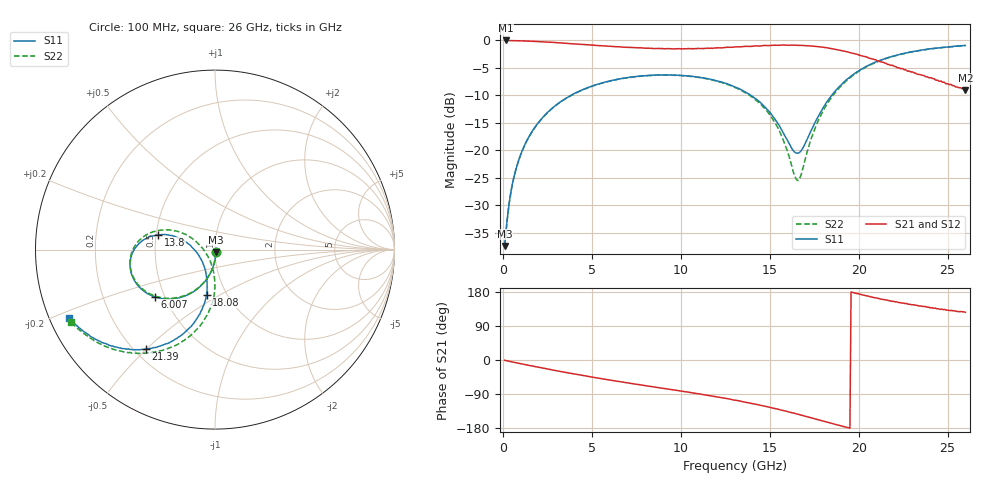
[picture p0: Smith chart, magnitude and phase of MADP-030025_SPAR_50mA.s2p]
!Mean
# HZ S DB R 50
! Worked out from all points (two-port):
!   400 points, 100 MHz to 26 GHz, reference 50 ohm
!   highest |S21| = -0.03 dB at 164.9 MHz (marker M1); lowest = -9.1 dB at 26 GHz (marker M2)
!   |S21| within 3 dB of the highest: start of sweep to 20.44 GHz
!   lowest |S11| = -37.4 dB at 100 MHz (marker M3), VSWR 1.03, Z = 50.4 - j1.29 ohm
!   |S11| at or under -10 dB: start of sweep to 3.835 GHz; 13.94 GHz to 18.49 GHz (4.546 GHz wide, 28 % of centre)
!   |S22| runs from -37.4 to -0.9 dB; largest |S21 - S12| = 0.0063
!   S11 on the Smith chart (normalised r, x): 100 MHz: 1.01, -0.03; 6.007 GHz: 0.44, -0.28; 13.8 GHz: 0.51, +0.09; 18.08 GHz: 0.81, -0.43; 21.39 GHz: 0.25, -0.50; 26 GHz: 0.06, -0.22
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1e8  -37.38 -71.7  -0.04 -0.8  -0.04 -0.8  -37.41 -71.7
1.6491e8  -35.34 -76.2  -0.03 -1.6  -0.04 -1.5  -35.26 -76.8
3.5965e8  -29.53 -84.0  -0.05 -3.5  -0.05 -3.5  -29.55 -84.1
5.5439e8  -25.86 -88.6  -0.06 -5.4  -0.07 -5.4  -25.93 -88.4
1.3333e9  -18.32 -99.5  -0.13 -12.9  -0.14 -12.9  -18.38 -99.6
2.6316e9  -12.75 -112.9  -0.34 -24.9  -0.34 -24.9  -12.79 -113.3
4.4491e9  -9.03 -129.4  -0.75 -40.6  -0.75 -40.6  -9.06 -130.0
6.007e9  -7.40 -142.0  -1.09 -53.0  -1.10 -53.0  -7.42 -142.8
8.7982e9  -6.30 -162.3  -1.47 -73.3  -1.48 -73.3  -6.34 -163.7
1.1005e10  -6.69 -177.1  -1.47 -89.1  -1.47 -89.1  -6.74 -179.5
1.3082e10  -8.52 169.3  -1.20 -106.2  -1.22 -106.2  -8.62 165.3
1.3796e10  -9.70 165.4  -1.11 -112.6  -1.11 -112.7  -9.85 160.3
1.5419e10  -14.90 164.0  -0.90 -129.3  -0.90 -129.4  -15.64 152.9
1.6523e10  -20.52 -153.2  -0.92 -142.3  -0.91 -142.4  -25.39 -156.9
1.6782e10  -20.02 -133.2  -0.92 -145.5  -0.93 -145.4  -24.29 -121.0
1.7367e10  -16.16 -107.7  -1.04 -152.8  -1.04 -152.7  -17.57 -92.8
1.8081e10  -11.85 -100.7  -1.31 -162.0  -1.31 -162.0  -12.34 -90.7
1.9379e10  -6.99 -107.1  -2.10 -178.2  -2.09 -178.2  -7.15 -101.4
2.1391e10  -3.42 -124.7  -4.01 159.7  -4.00 159.9  -3.49 -121.2
2.1716e10  -3.08 -127.3  -4.39 156.5  -4.38 156.5  -3.14 -124.1
2.4053e10  -1.54 -144.1  -6.78 137.7  -6.74 138.2  -1.55 -141.8
2.6e10  -0.94 -154.7  -9.10 125.9  -8.96 125.8  -0.94 -153.1
